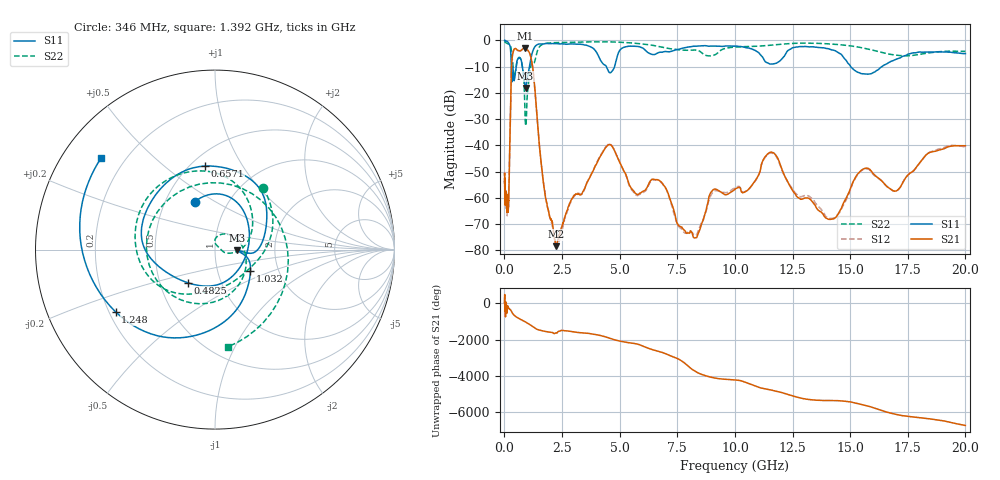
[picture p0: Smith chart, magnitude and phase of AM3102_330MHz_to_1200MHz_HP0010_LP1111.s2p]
! Date/Time: Tue, Sep 11, 2018 5:11 PM
! Network Analyzer: Agilent Technologies E8362B Rev: A.07.50.63
! Sweep from 0.010 to 20.000 GHz, 1601 Points, Sweep Type: LOG
! Power Supply: 4.950 V, 0.001 A
# Hz S DB R 50
!freq MagS11 AngS11 MagS21 AngS21 MagS12 AngS12 MagS22 AngS22
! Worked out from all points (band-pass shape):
!   1601 points, 10 MHz to 20 GHz, reference 50 ohm
!   highest |S21| = -2.98 dB at 886.4 MHz (marker M1); lowest = -78.4 dB at 2.238 GHz (marker M2)
!   |S21| within 3 dB of the highest: 345.6 MHz to 1.138 GHz (792.3 MHz wide, 107 % of centre)
!   lowest |S11| = -18.1 dB at 920.7 MHz (marker M3), VSWR 1.28, Z = 64.2 - j0.605 ohm
!   |S11| at or under -10 dB: 780.8 MHz to 1.087 GHz (305.8 MHz wide, 32.8 % of centre); 4.427 GHz to 4.78 GHz (352.9 MHz wide, 7.67 % of centre); 15.03 GHz to 16.37 GHz (1.345 GHz wide, 8.57 % of centre)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
!   |S22| runs from -32.5 to -0.3 dB; largest |S21 - S12| = 0.013
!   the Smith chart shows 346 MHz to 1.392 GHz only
!   S11 on the Smith chart (normalised r, x): 346 MHz: 0.70, +0.41; 482.5 MHz: 0.69, -0.27; 657.1 MHz: 0.59, +0.70; 1.032 GHz: 1.44, -0.37; 1.248 GHz: 0.23, -0.27; 1.392 GHz: 0.11, +0.35
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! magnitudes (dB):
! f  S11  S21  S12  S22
! 10 MHz  0.0  -51.2  -51.0  -0.3
! 35.55 MHz  0.0  -61.5  -61.1  -0.6
! 126.4 MHz  -0.4  -64.2  -65.0  -1.1
! 187.5 MHz  -1.1  -60.2  -60.1  -1.4
! 346 MHz  -10.8  -6.0  -6.0  -7.2
! 447.2 MHz  -14.3  -3.1  -3.2  -13.6
! 482.5 MHz  -12.4  -3.1  -3.1  -12.1
! 657.1 MHz  -6.6  -3.9  -4.1  -6.5
! 886.4 MHz  -16.8  -3.0  -3.0  -24.9
! 920.7 MHz  -18.1  -3.0  -3.1  -32.3
! 1.032 GHz  -12.7  -3.9  -3.9  -17.3
! 1.248 GHz  -3.7  -11.6  -11.7  -8.5
! 1.392 GHz  -1.8  -26.0  -26.4  -5.2
! 1.59 GHz  -1.3  -46.2  -46.2  -1.8
! 2.238 GHz  -1.2  -78.4  -77.7  -0.8
! 4.479 GHz  -11.0  -40.1  -39.8  -0.5
! 5.652 GHz  -2.2  -57.9  -58.3  -1.0
! 6.739 GHz  -4.5  -53.5  -53.6  -2.4
! 8.188 GHz  -2.2  -74.8  -73.6  -3.6
! 11.58 GHz  -9.0  -42.5  -42.9  -1.8
! 14.07 GHz  -3.2  -68.2  -67.7  -1.3
! 20 GHz  -5.0  -40.1  -40.6  -4.2
